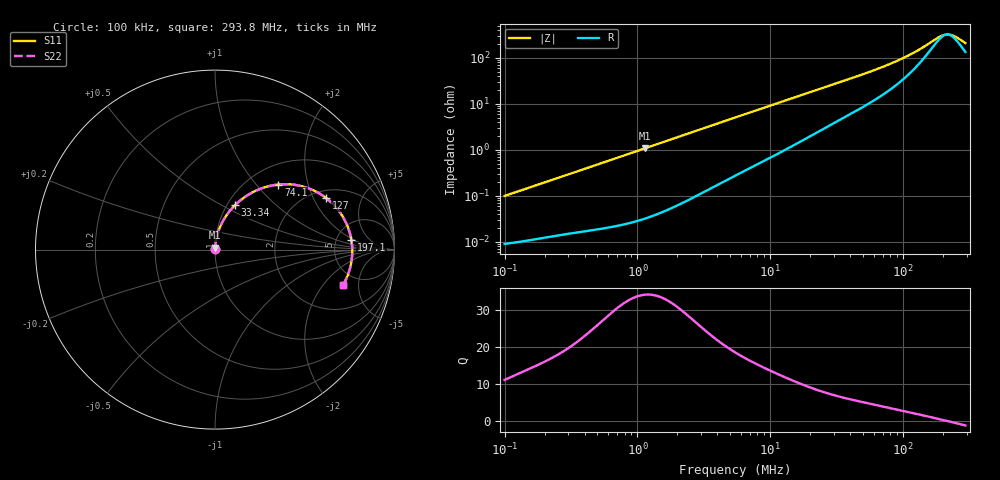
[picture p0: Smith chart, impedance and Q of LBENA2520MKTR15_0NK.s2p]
! LBENA2520MKTR15_0NK  S-PARAMETER MODEL  ( General Type )
! Model Generated by TAIYO YUDEN Corporation (http://www.ty-top.com)
! Version 1.0
! TAIYO YUDEN Control No. 220120
! Copyright(c) 2022 TAIYO YUDEN CO.,LTD. All Rights Reserved.
! Product Description (link to TY-COMPAS)
! https://ds.yuden.co.jp/TYCOMPAS/or/detail?pn=LBENA2520MKTR15M0NK&u=M
! Products Name : Inductors
! Characteristics :
!  Inductance : 0.15 uH , SRF(min) : -Hz , DC Resistance(max) : 0.009 Ohm
!  Rated Current : Saturation :10200 mA , Temp Rise : 6700 mA
!  Case Size : 2.5 x 2.0 / 0.098 x 0.079 [mm/inch] , Thickness : 1.2 / 0.047 [mm/inch]
!  (Conditions: Temperature = 25 degC , DC Bias Current/Voltage = 0A / 0V)
! External Node Assignments :
!  1  o---GGG---o  2
! GND o---------o GND
! Frequency Range : 0.1MHz  -  293.796821MHz  [ 402 STEP ]
# MHz S RI R 50
! Freq[MHz].  S11 Real  S11 Imag  S21 Real  S21 Imag  S12 Real  S12 Imag  S22 Real  S22 Imag
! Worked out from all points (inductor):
!   401 points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, 100 kHz to 293.8 MHz, reference 50 ohm
!   read as one part in series: L = 157 nH near 104.1 kHz
!   highest Q = 34 at 1.142 MHz (marker M1), where L = 151 nH
!   self-resonance near 214.6 MHz
!   S11 on the Smith chart (normalised r, x): 100 kHz: 1.00, +0.00; 33.34 MHz: 1.09, +0.58; 74.1 MHz: 1.35, +1.32; 127 MHz: 2.34, +2.52; 197.1 MHz: 6.88, +1.84; 293.8 MHz: 3.70, -3.26
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0.1  9.04e-05 0.000989  0.9999 -0.000989  0.9999 -0.000989  9.04e-05 0.000989
0.380976  0.000178 0.00366  0.9998 -0.00366  0.9998 -0.00366  0.000178 0.00366
1.142232  0.000437 0.0108  0.9996 -0.0108  0.9996 -0.0108  0.000437 0.0108
1.451429  0.0006 0.0138  0.9994 -0.0138  0.9994 -0.0138  0.0006 0.0138
5.420303  0.00523 0.05  0.9948 -0.05  0.9948 -0.05  0.00523 0.05
10.90128  0.0172 0.0969  0.9828 -0.0969  0.9828 -0.0969  0.0172 0.0969
20.65007  0.0514 0.1713  0.9486 -0.1713  0.9486 -0.1713  0.0514 0.1713
33.34297  0.1124 0.2484  0.8876 -0.2484  0.8876 -0.2484  0.1124 0.2484
41.5313  0.1574 0.2868  0.8426 -0.2868  0.8426 -0.2868  0.1574 0.2868
50.70803  0.2111 0.3202  0.7889 -0.3202  0.7889 -0.3202  0.2111 0.3202
60.68869  0.2716 0.3455  0.7284 -0.3455  0.7284 -0.3455  0.2716 0.3455
74.09842  0.3531 0.3626  0.6469 -0.3626  0.6469 -0.3626  0.3531 0.3626
78.67184  0.3804 0.3644  0.6196 -0.3644  0.6196 -0.3644  0.3804 0.3644
99.96794  0.4985 0.3489  0.5015 -0.3489  0.5015 -0.3489  0.4985 0.3489
127.0288  0.6184 0.2881  0.3816 -0.2881  0.3816 -0.2881  0.6184 0.2881
161.4149  0.7154 0.1776  0.2846 -0.1776  0.2846 -0.1776  0.7154 0.1776
181.9551  0.7468 0.1069  0.2532 -0.1069  0.2532 -0.1069  0.7468 0.1069
197.081  0.7594 0.0561  0.2406 -0.0561  0.2406 -0.0561  0.7594 0.0561
213.4643  0.7647 0.00347  0.2353 -0.00347  0.2353 -0.00347  0.7647 0.00347
231.2095  0.7626 -0.0496  0.2374 0.0496  0.2374 0.0496  0.7626 -0.0496
250.4299  0.753 -0.1018  0.247 0.1018  0.247 0.1018  0.753 -0.1018
293.7968  0.7127 -0.199  0.2873 0.199  0.2873 0.199  0.7127 -0.199
